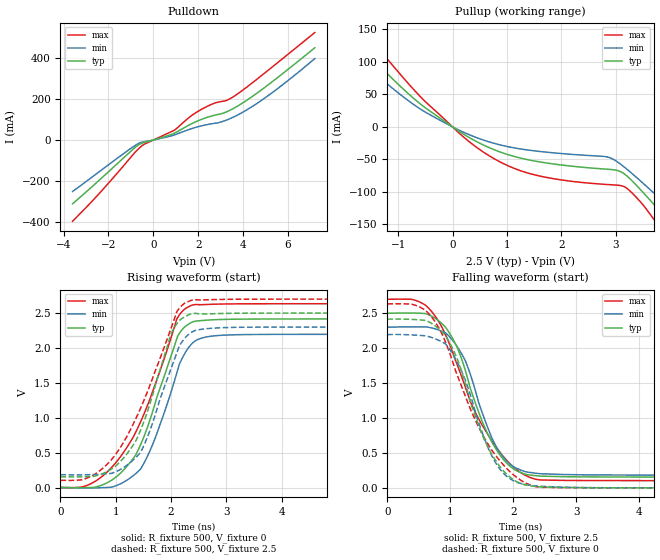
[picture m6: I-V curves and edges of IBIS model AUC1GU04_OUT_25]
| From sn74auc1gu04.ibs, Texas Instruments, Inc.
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[Model]   AUC1GU04_OUT_25
Model_type  Output
Vref =   0
Rref =   500
Cref =   30p
Vmeas =   1.25
| variable   typ   min   max
C_comp   3.99pF   2.71pF   5.27pF
| C_pullup   3.81pF   2.71pF   4.70pF
| C_pulldown   4.16pF   3.46pF   5.27pF
[Temperature Range]   40   100   -40
| Ambient temperature   25   85   -40
[Voltage range]   2.5   2.3   2.7
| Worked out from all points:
|   slope of the pulldown table from 0 to 0.375 V, typ, clamps not added: 31 ohm
|   slope of the pullup table from 0 to 0.375 V, typ, clamps not added: 19.2 ohm
|   rising waveform, R_fixture 500, V_fixture 0: 20-80 % time 649ps typ, 578ps min, 823ps max; typ from 0 V to 2.42 V
|   falling waveform, R_fixture 500, V_fixture 2.5: 20-80 % time 582ps typ, 514ps min, 767ps max; typ from 2.5 V to 0.154 V
|   rising waveform, R_fixture 500, V_fixture 2.5: 20-80 % time 607ps typ, 569ps min, 833ps max; typ from 0.154 V to 2.5 V
|   falling waveform, R_fixture 500, V_fixture 0: 20-80 % time 589ps typ, 535ps min, 754ps max; typ from 2.42 V to 0 V
[Pulldown]
| AUC1GU04_OUT_25
|   Voltage   I(typ)   I(min)   I(max)
-3.6V     -310mA     -250.4mA   -395.2mA
-2.425V   -196.8mA   -155.2mA   -261.8mA
-1.07V    -61.46mA   -45.93mA   -92.26mA
-500mV    -15.26mA   -10.33mA   -27.19mA
940mV     33.3mA     24.95mA    48.08mA
1.675V    77.37mA    54.21mA    116.3mA
2.21V     102.8mA    70.5mA     152.9mA
2.985V    126.7mA    86.79mA    186.4mA
3.275V    137.4mA    97.56mA    193.3mA
3.62V     156.3mA    114mA      214.1mA
5.105V    267.1mA    214.6mA    337.8mA
7.2V      448.7mA    395.9mA    522.6mA
[Pullup]
| AUC1GU04_OUT_25
|   Voltage   I(typ)   I(min)   I(max)
-3.6V     294.7mA    268mA      329.7mA
-2.39V    185.6mA    159.9mA    219.7mA
-1.965V   147.7mA    124.4mA    179.1mA
-1.705V   124.8mA    103.7mA    153.9mA
-610mV    36.49mA    28.44mA    48.1mA
585mV     -28.48mA   -20.67mA   -39.69mA
1.51V     -52.44mA   -36.81mA   -73.66mA
3.05V     -67.49mA   -54.83mA   -89.69mA
3.28V     -81.08mA   -70.23mA   -99.81mA
3.85V     -133mA     -113mA     -159.2mA
4.39V     -184.3mA   -155.3mA   -221.5mA
7.2V      -450.3mA   -380.1mA   -537.9mA
[Ramp]
| AUC1GU04_OUT_25
| variable   typ   min   max
dV/dt_r   1.45/6.50E-10   1.32/6.03E-10   1.58/8.37E-10
dV/dt_f   1.41/5.92E-10   1.27/5.43E-10   1.56/7.88E-10
R_load = 500
[Rising Waveform]
| AUC1GU04_OUT_25
R_fixture =   500
C_fixture =   0
L_fixture =   0
V_fixture =   0
V_fixture_min = 0
V_fixture_max = 0
|   Time   V(typ)   V(min)   V(max)
0s        4.69nV     6.22nV     324.6nV
760ps     37.51mV    -1.794mV   162.9mV
1.135ns   244.6mV    72.89mV    495.8mV
1.445ns   604.4mV    260.4mV    932.7mV
1.72ns    1.227V     722.6mV    1.492V
2.105ns   2.132V     1.642V     2.416V
2.245ns   2.3V       1.915V     2.555V
2.435ns   2.384V     2.1V       2.622V
3.76ns    2.415V     2.195V     2.634V
34.99ns   2.416V     2.195V     2.634V
[Falling Waveform]
| AUC1GU04_OUT_25
R_fixture =   500
C_fixture =   0
L_fixture =   0
V_fixture =   2.5
V_fixture_min = 2.3
V_fixture_max = 2.7
|   Time   V(typ)   V(min)   V(max)
0s        2.5V       2.3V       2.7V
605ps     2.496V     2.305V     2.616V
950ps     2.267V     2.198V     2.14V
1.12ns    1.989V     2.007V     1.737V
1.24ns    1.675V     1.816V     1.441V
1.51ns    942.6mV    1.068V     891.7mV
1.735ns   541.1mV    582mV      573.6mV
2.005ns   270.2mV    300.9mV    297.9mV
2.435ns   167.9mV    202.2mV    112.7mV
34.99ns   154.5mV    183.4mV    103.3mV
[Rising Waveform]
| AUC1GU04_OUT_25
R_fixture =   500
C_fixture =   0
L_fixture =   0
V_fixture =   2.5
V_fixture_min = 2.3
V_fixture_max = 2.7
|   Time   V(typ)   V(min)   V(max)
0s        154.5mV    183.4mV    103.3mV
425ps     154.4mV    182.4mV    119.8mV
775ps     203.3mV    192.7mV    282mV
1.105ns   390.3mV    268.2mV    601mV
1.415ns   756.7mV    472.6mV    1.075V
1.605ns   1.165V     787.3mV    1.437V
2.005ns   2.205V     1.712V     2.292V
2.155ns   2.394V     2.034V     2.573V
2.425ns   2.496V     2.247V     2.691V
34.99ns   2.5V       2.3V       2.7V
[Falling Waveform]
| AUC1GU04_OUT_25
R_fixture =   500
C_fixture =   0
L_fixture =   0
V_fixture =   0
V_fixture_min = 0
V_fixture_max = 0
|   Time   V(typ)   V(min)   V(max)
0s        2.416V     2.195V     2.634V
600ps     2.398V     2.178V     2.545V
775ps     2.31V      2.129V     2.354V
925ps     2.177V     2.059V     2.086V
1.21ns    1.583V     1.606V     1.38V
1.45ns    894.6mV    936.3mV    871.4mV
1.695ns   426.2mV    397.7mV    494mV
1.995ns   120.8mV    105.8mV    192.4mV
2.425ns   13.59mV    23.2mV     8.585mV
34.99ns   30.25nV    57.45nV    347.7nV
